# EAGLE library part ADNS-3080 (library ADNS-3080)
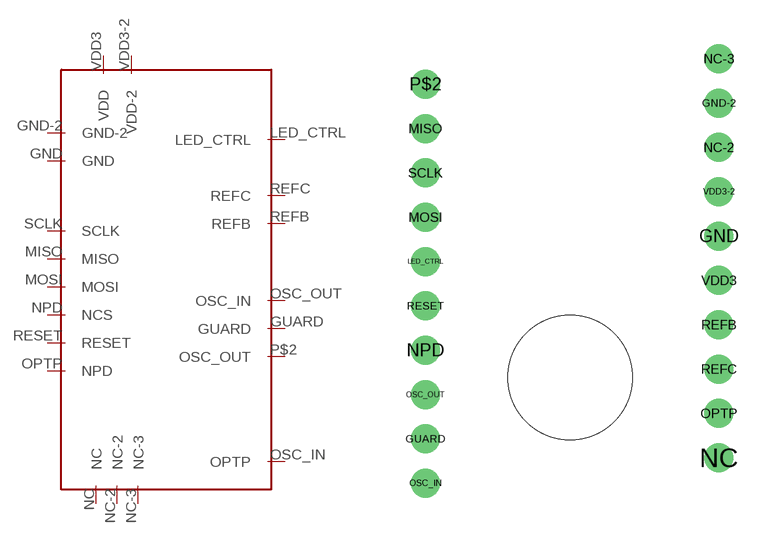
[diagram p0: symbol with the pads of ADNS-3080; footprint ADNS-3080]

Designator prefix -

## ADNS-3080  [ADNS-3080]
GND  GND
GND-2  GND-2
GUARD  GUARD
LED_CTRL  LED_CTRL
MISO  MISO
MOSI  MOSI
NC  NC
NC-2  NC-2
NC-3  NC-3
NPD  NCS
OPTP  NPD
OSC_IN  OPTP
OSC_OUT  OSC_IN
P$2  OSC_OUT
REFB  REFB
REFC  REFC
RESET  RESET
SCLK  SCLK
VDD3  VDD
VDD3-2  VDD-2

## Footprint ADNS-3080 (pad centres in mm)
drill 0.8: GND 6.72,6.38; GND-2 6.72,12.38; GUARD -6.53,-2.77; LED_CTRL -6.53,5.23; MISO -6.53,11.23; MOSI -6.53,7.23; NC 6.72,-3.62; NC-2 6.72,10.38; NC-3 6.72,14.38; NPD -6.53,1.23; OPTP 6.72,-1.62; OSC_IN -6.53,-4.77; OSC_OUT -6.53,-0.77; P$2 -6.53,13.23; REFB 6.72,2.38; REFC 6.72,0.38; RESET -6.53,3.23; SCLK -6.53,9.23; VDD3 6.72,4.38; VDD3-2 6.72,8.38
hole 5.6 at 0,0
